(* Logix 5000 AddOnInstructionDefinition export Banner_Q20EAF_Param_v4; software revision 33.00; part 2 of 2 *)
(* tags used below, declared in another part *)
   Q20 : Banner_Q20EAF_v4;
   Port_Data : Banner_IOL_Port_v4;
   Port : DINT;
   Local_Control : DINT;
   Command_Being_Processed : BOOL;
   Update_Archive : BOOL;
   Index_Write_Inprocess : INT;
   Index_Write_Control : INT;
   Inprocess_Index : DINT;
(* Banner_Q20EAF_Param_v4, continued *)

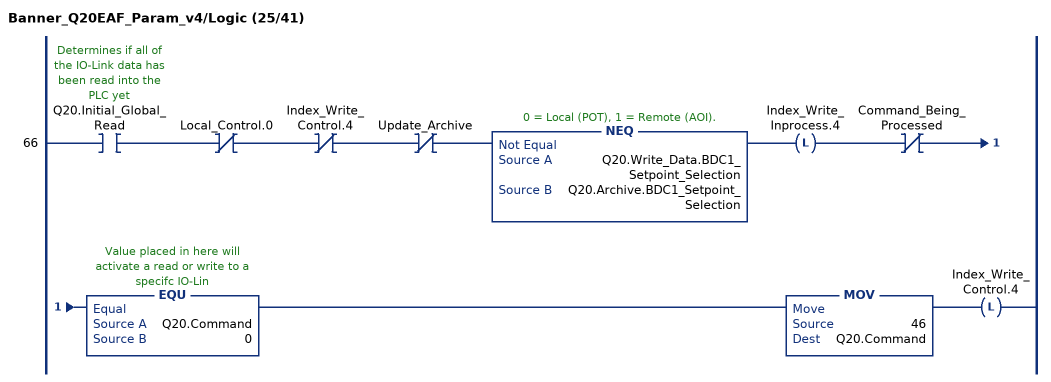
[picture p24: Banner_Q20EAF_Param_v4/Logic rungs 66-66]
   66: XIC(Q20.Initial_Global_Read)XIO(Local_Control.0)XIO(Index_Write_Control.4)XIO(Update_Archive)NEQ(Q20.Write_Data.BDC1_Setpoint_Selection,Q20.Archive.BDC1_Setpoint_Selection)OTL(Index_Write_Inprocess.4)XIO(Command_Being_Processed)EQU(Q20.Command,0)MOV(46,Q20.Command)OTL(Index_Write_Control.4);
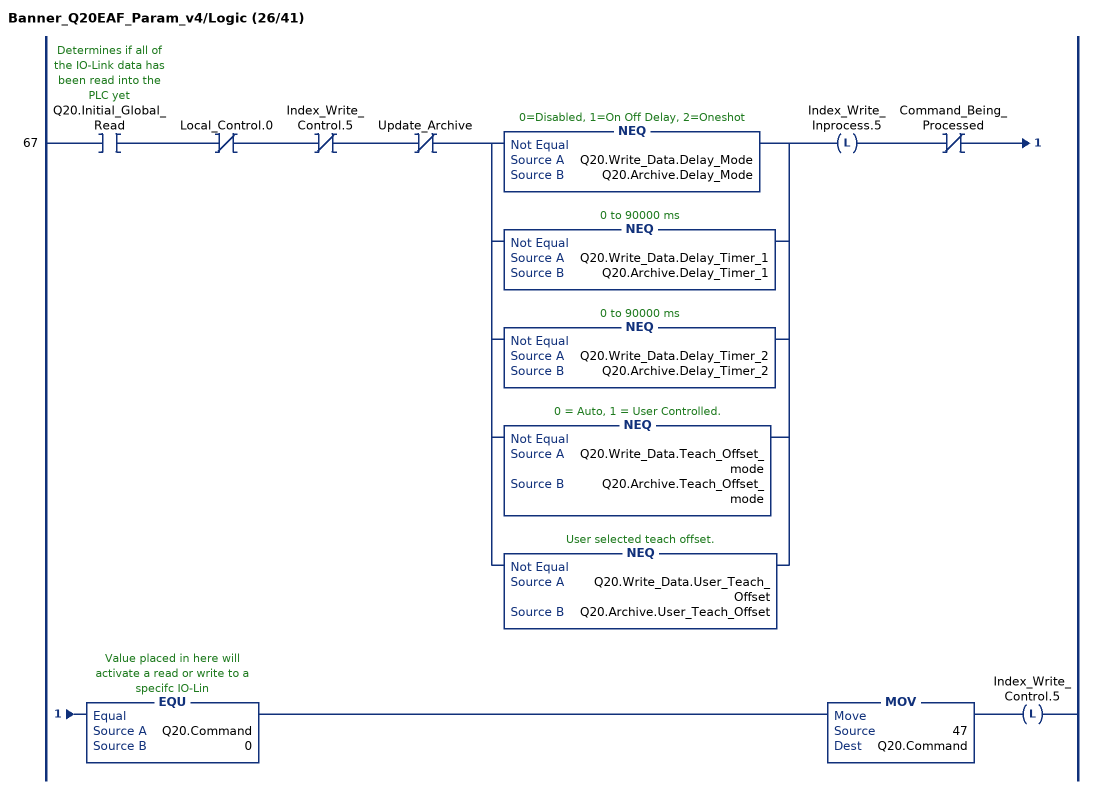
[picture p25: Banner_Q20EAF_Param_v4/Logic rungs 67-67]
   67: XIC(Q20.Initial_Global_Read)XIO(Local_Control.0)XIO(Index_Write_Control.5)XIO(Update_Archive)[NEQ(Q20.Write_Data.Delay_Mode,Q20.Archive.Delay_Mode) ,NEQ(Q20.Write_Data.Delay_Timer_1,Q20.Archive.Delay_Timer_1) ,NEQ(Q20.Write_Data.Delay_Timer_2,Q20.Archive.Delay_Timer_2) ,NEQ(Q20.Write_Data.Teach_Offset_mode,Q20.Archive.Teach_Offset_mode) ,NEQ(Q20.Write_Data.User_Teach_Offset,Q20.Archive.User_Teach_Offset) ]OTL(Index_Write_Inprocess.5)XIO(Command_Being_Processed)EQU(Q20.Command,0)MOV(47,Q20.Command)OTL(Index_Write_Control.5);
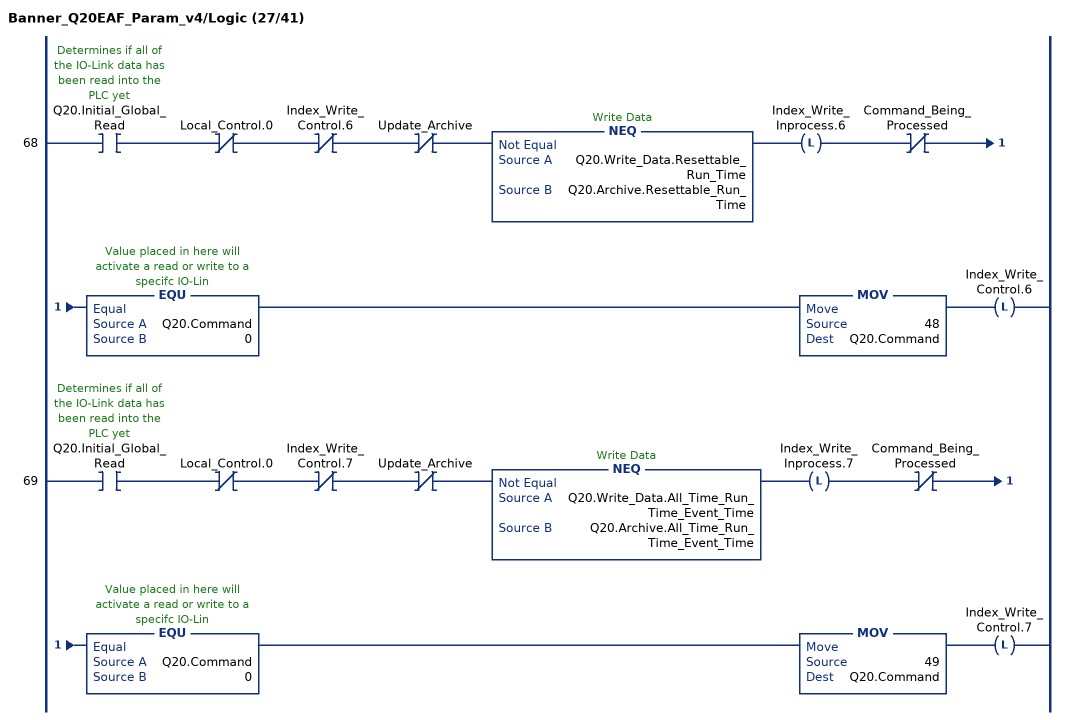
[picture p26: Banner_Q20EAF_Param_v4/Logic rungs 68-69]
   68: XIC(Q20.Initial_Global_Read)XIO(Local_Control.0)XIO(Index_Write_Control.6)XIO(Update_Archive)NEQ(Q20.Write_Data.Resettable_Run_Time,Q20.Archive.Resettable_Run_Time)OTL(Index_Write_Inprocess.6)XIO(Command_Being_Processed)EQU(Q20.Command,0)MOV(48,Q20.Command)OTL(Index_Write_Control.6);
   69: XIC(Q20.Initial_Global_Read)XIO(Local_Control.0)XIO(Index_Write_Control.7)XIO(Update_Archive)NEQ(Q20.Write_Data.All_Time_Run_Time_Event_Time,Q20.Archive.All_Time_Run_Time_Event_Time)OTL(Index_Write_Inprocess.7)XIO(Command_Being_Processed)EQU(Q20.Command,0)MOV(49,Q20.Command)OTL(Index_Write_Control.7);
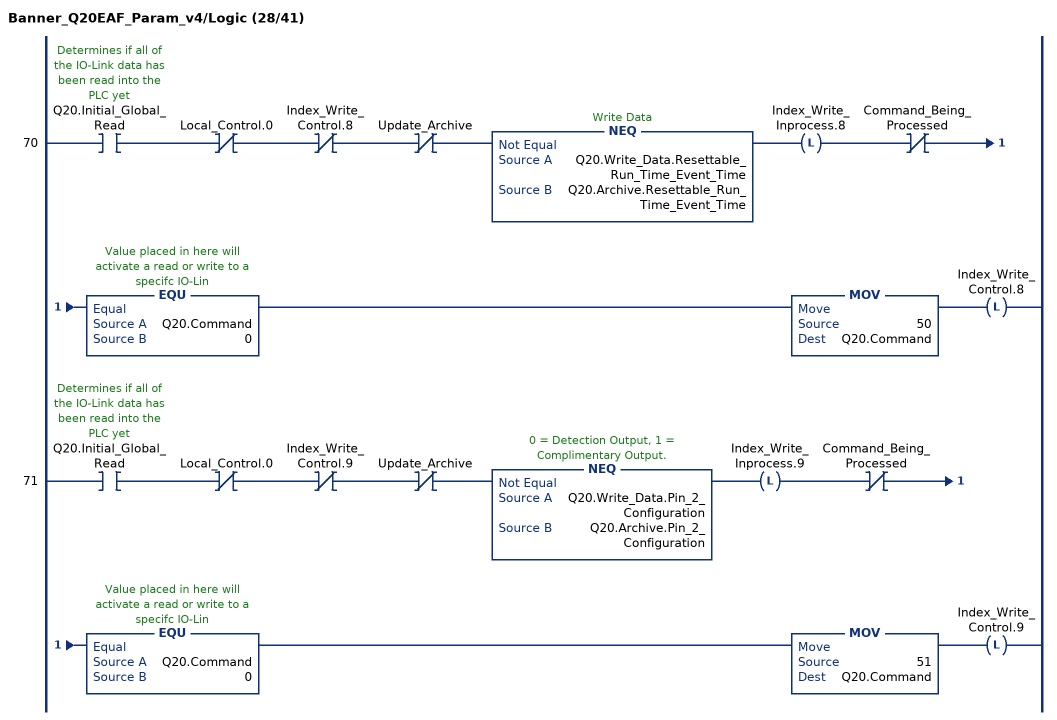
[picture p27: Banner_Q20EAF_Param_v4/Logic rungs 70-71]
   70: XIC(Q20.Initial_Global_Read)XIO(Local_Control.0)XIO(Index_Write_Control.8)XIO(Update_Archive)NEQ(Q20.Write_Data.Resettable_Run_Time_Event_Time,Q20.Archive.Resettable_Run_Time_Event_Time)OTL(Index_Write_Inprocess.8)XIO(Command_Being_Processed)EQU(Q20.Command,0)MOV(50,Q20.Command)OTL(Index_Write_Control.8);
   71: XIC(Q20.Initial_Global_Read)XIO(Local_Control.0)XIO(Index_Write_Control.9)XIO(Update_Archive)NEQ(Q20.Write_Data.Pin_2_Configuration,Q20.Archive.Pin_2_Configuration)OTL(Index_Write_Inprocess.9)XIO(Command_Being_Processed)EQU(Q20.Command,0)MOV(51,Q20.Command)OTL(Index_Write_Control.9);
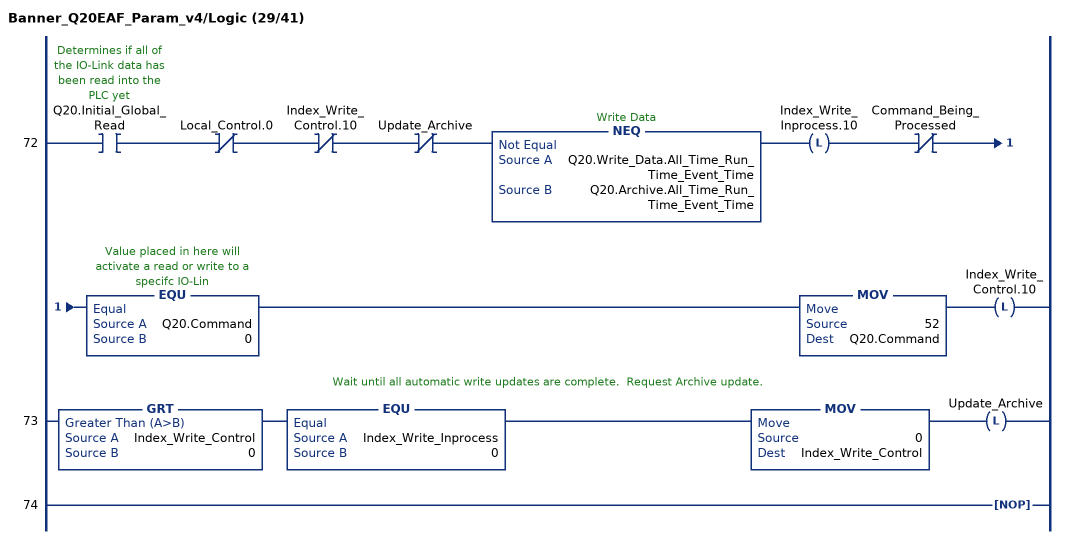
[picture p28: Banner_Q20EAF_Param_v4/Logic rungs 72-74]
   72: XIC(Q20.Initial_Global_Read)XIO(Local_Control.0)XIO(Index_Write_Control.10)XIO(Update_Archive)NEQ(Q20.Write_Data.All_Time_Run_Time_Event_Time,Q20.Archive.All_Time_Run_Time_Event_Time)OTL(Index_Write_Inprocess.10)XIO(Command_Being_Processed)EQU(Q20.Command,0)MOV(52,Q20.Command)OTL(Index_Write_Control.10);
   // Wait until all automatic write updates are complete.  Request Archive update.
   73: GRT(Index_Write_Control,0)EQU(Index_Write_Inprocess,0)MOV(0,Index_Write_Control)OTL(Update_Archive);
   74: NOP();
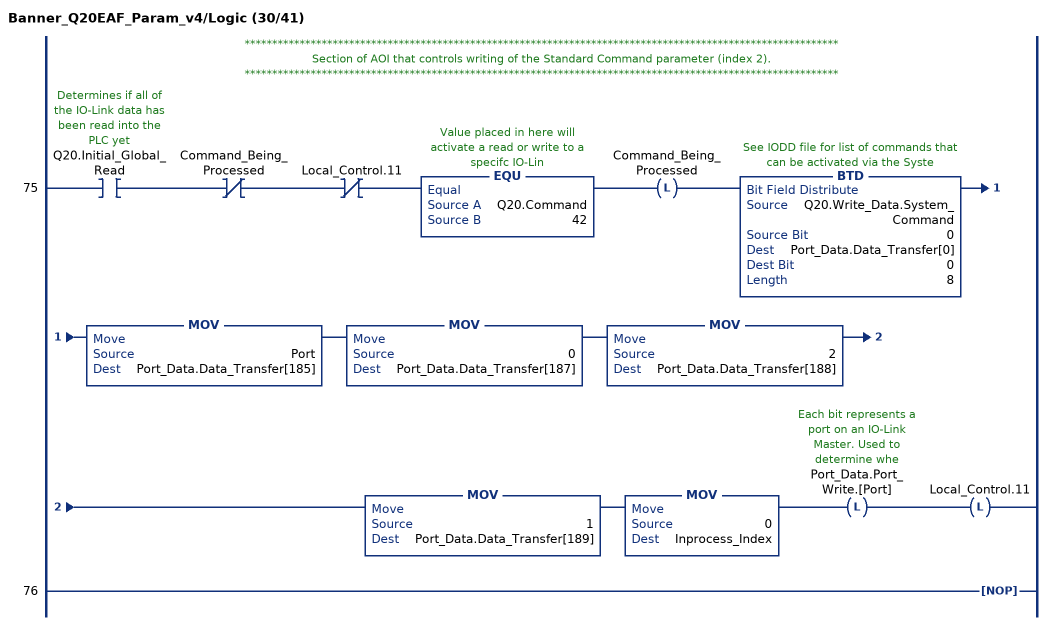
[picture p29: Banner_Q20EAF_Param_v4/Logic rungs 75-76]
   // ************************************************************************************************************
   // Section of AOI that controls writing of the Standard Command parameter (index 2).
   // ************************************************************************************************************
   75: XIC(Q20.Initial_Global_Read)XIO(Command_Being_Processed)XIO(Local_Control.11)EQU(Q20.Command,42)OTL(Command_Being_Processed)BTD(Q20.Write_Data.System_Command,0,Port_Data.Data_Transfer[0],0,8)MOV(Port,Port_Data.Data_Transfer[185])MOV(0,Port_Data.Data_Transfer[187])MOV(2,Port_Data.Data_Transfer[188])MOV(1,Port_Data.Data_Transfer[189])MOV(0,Inprocess_Index)OTL(Port_Data.Port_Write.[Port])OTL(Local_Control.11);
   76: NOP();
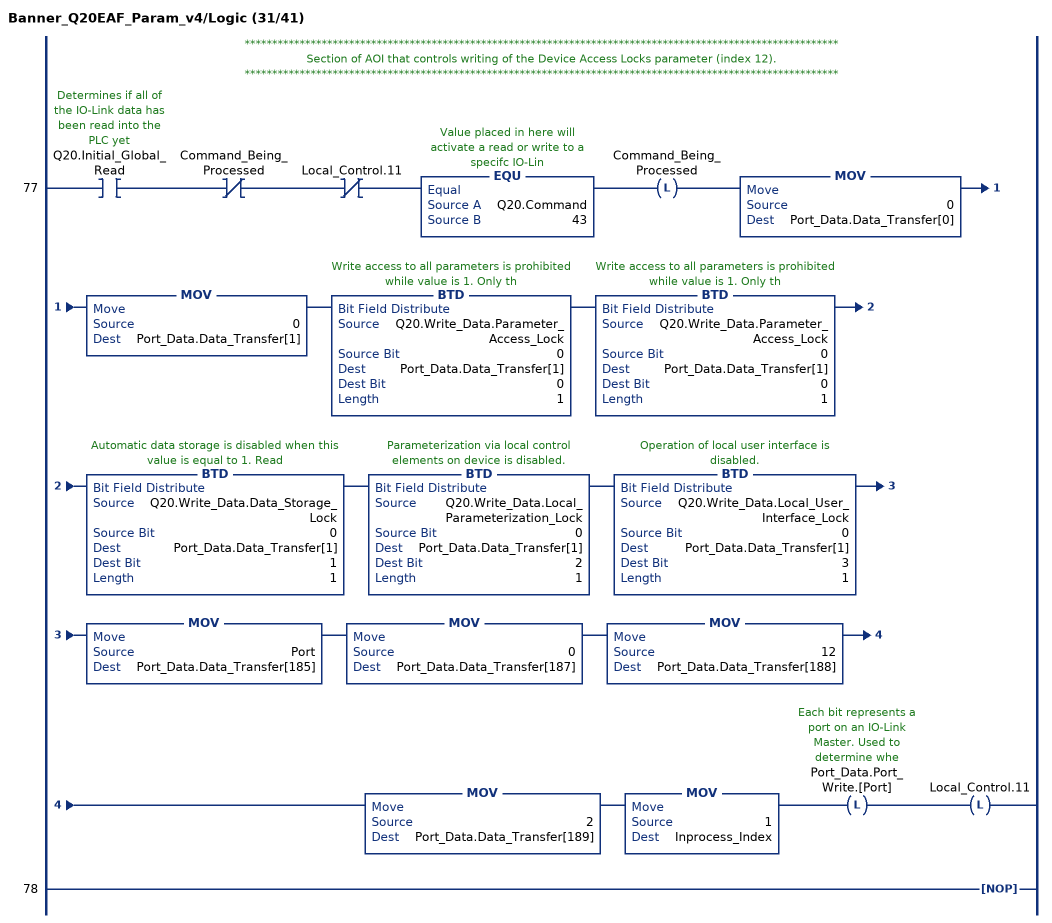
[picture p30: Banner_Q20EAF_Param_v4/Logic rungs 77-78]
   // ************************************************************************************************************
   // Section of AOI that controls writing of the Device Access Locks parameter (index 12).
   // ************************************************************************************************************
   77: XIC(Q20.Initial_Global_Read)XIO(Command_Being_Processed)XIO(Local_Control.11)EQU(Q20.Command,43)OTL(Command_Being_Processed)MOV(0,Port_Data.Data_Transfer[0])MOV(0,Port_Data.Data_Transfer[1])BTD(Q20.Write_Data.Parameter_Access_Lock,0,Port_Data.Data_Transfer[1],0,1)BTD(Q20.Write_Data.Parameter_Access_Lock,0,Port_Data.Data_Transfer[1],0,1)BTD(Q20.Write_Data.Data_Storage_Lock,0,Port_Data.Data_Transfer[1],1,1)BTD(Q20.Write_Data.Local_Parameterization_Lock,0,Port_Data.Data_Transfer[1],2,1)BTD(Q20.Write_Data.Local_User_Interface_Lock,0,Port_Data.Data_Transfer[1],3,1)MOV(Port,Port_Data.Data_Transfer[185])MOV(0,Port_Data.Data_Transfer[187])MOV(12,Port_Data.Data_Transfer[188])MOV(2,Port_Data.Data_Transfer[189])MOV(1,Inprocess_Index)OTL(Port_Data.Port_Write.[Port])OTL(Local_Control.11);
   78: NOP();
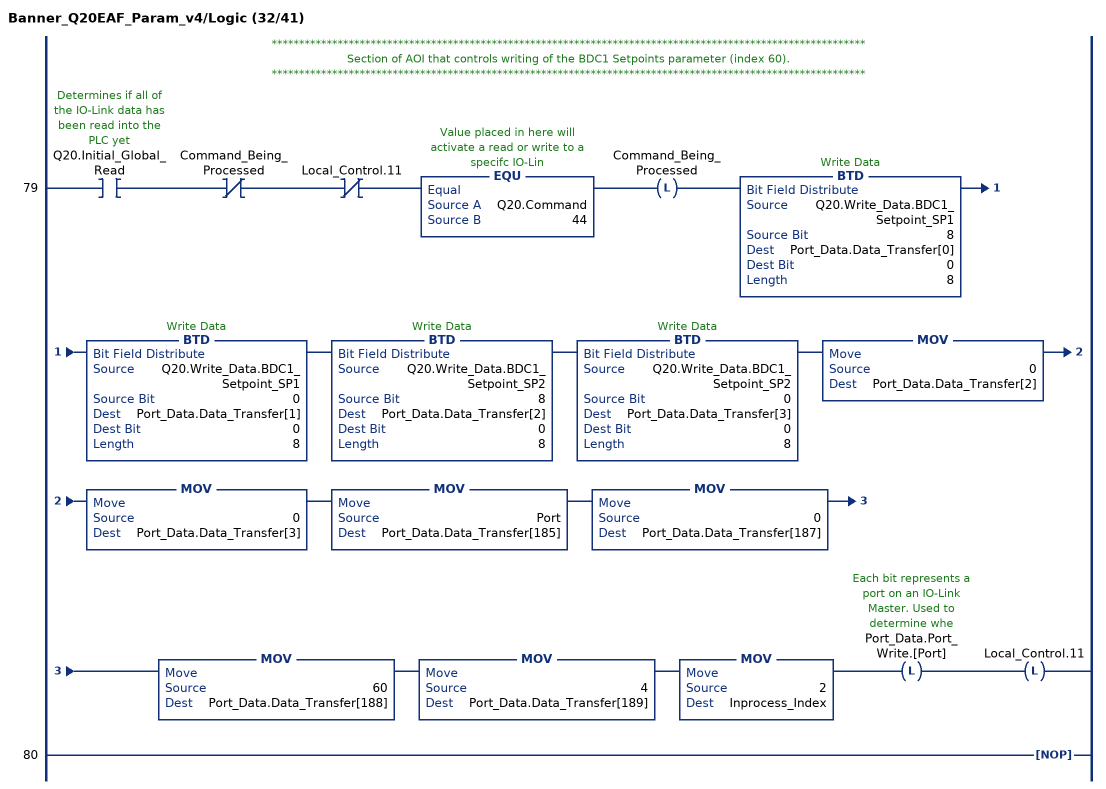
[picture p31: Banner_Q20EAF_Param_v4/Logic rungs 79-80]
   // ************************************************************************************************************
   // Section of AOI that controls writing of the BDC1 Setpoints parameter (index 60).
   // ************************************************************************************************************
   79: XIC(Q20.Initial_Global_Read)XIO(Command_Being_Processed)XIO(Local_Control.11)EQU(Q20.Command,44)OTL(Command_Being_Processed)BTD(Q20.Write_Data.BDC1_Setpoint_SP1,8,Port_Data.Data_Transfer[0],0,8)BTD(Q20.Write_Data.BDC1_Setpoint_SP1,0,Port_Data.Data_Transfer[1],0,8)BTD(Q20.Write_Data.BDC1_Setpoint_SP2,8,Port_Data.Data_Transfer[2],0,8)BTD(Q20.Write_Data.BDC1_Setpoint_SP2,0,Port_Data.Data_Transfer[3],0,8)MOV(0,Port_Data.Data_Transfer[2])MOV(0,Port_Data.Data_Transfer[3])MOV(Port,Port_Data.Data_Transfer[185])MOV(0,Port_Data.Data_Transfer[187])MOV(60,Port_Data.Data_Transfer[188])MOV(4,Port_Data.Data_Transfer[189])MOV(2,Inprocess_Index)OTL(Port_Data.Port_Write.[Port])OTL(Local_Control.11);
   80: NOP();
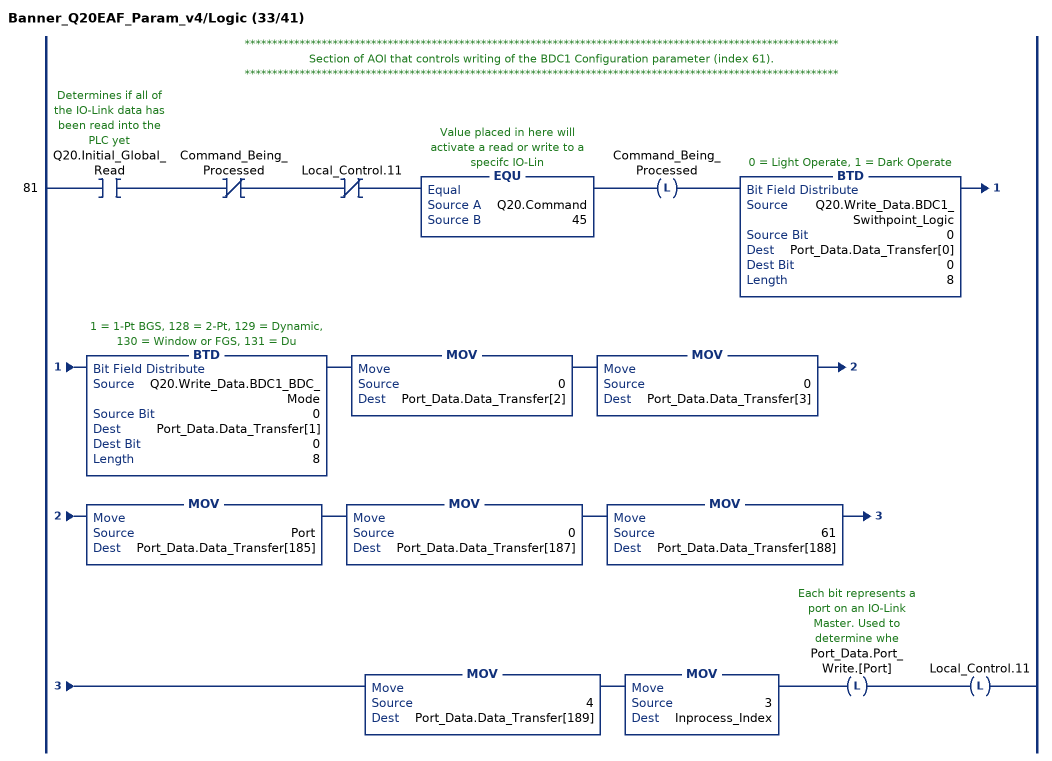
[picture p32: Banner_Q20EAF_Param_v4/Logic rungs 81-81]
   // ************************************************************************************************************
   // Section of AOI that controls writing of the BDC1 Configuration parameter (index 61).
   // ************************************************************************************************************
   81: XIC(Q20.Initial_Global_Read)XIO(Command_Being_Processed)XIO(Local_Control.11)EQU(Q20.Command,45)OTL(Command_Being_Processed)BTD(Q20.Write_Data.BDC1_Swithpoint_Logic,0,Port_Data.Data_Transfer[0],0,8)BTD(Q20.Write_Data.BDC1_BDC_Mode,0,Port_Data.Data_Transfer[1],0,8)MOV(0,Port_Data.Data_Transfer[2])MOV(0,Port_Data.Data_Transfer[3])MOV(Port,Port_Data.Data_Transfer[185])MOV(0,Port_Data.Data_Transfer[187])MOV(61,Port_Data.Data_Transfer[188])MOV(4,Port_Data.Data_Transfer[189])MOV(3,Inprocess_Index)OTL(Port_Data.Port_Write.[Port])OTL(Local_Control.11);
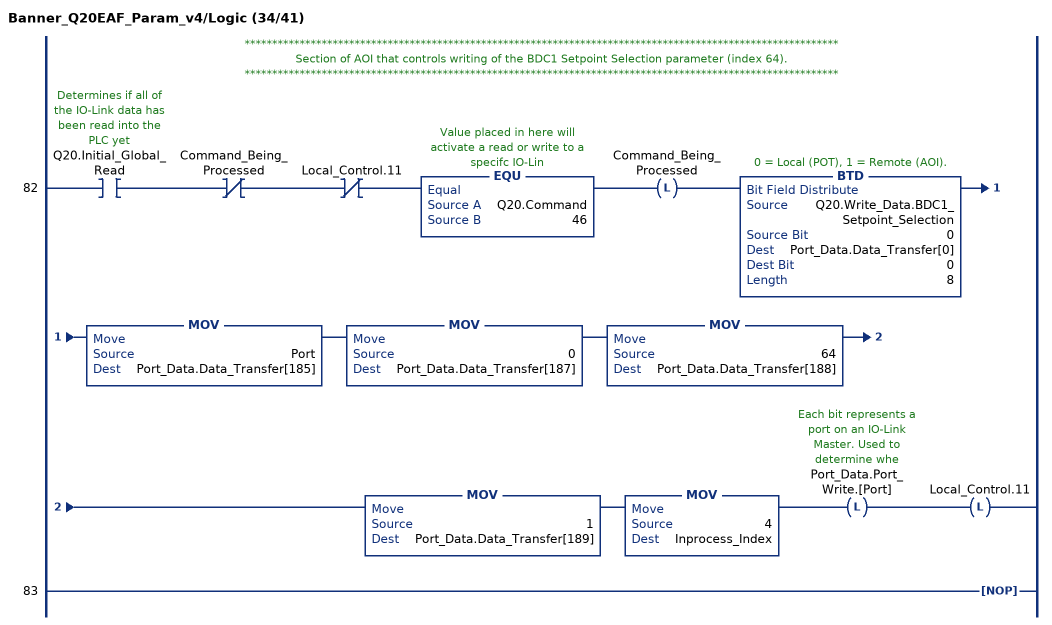
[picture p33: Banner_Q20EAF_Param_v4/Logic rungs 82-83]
   // ************************************************************************************************************
   // Section of AOI that controls writing of the BDC1 Setpoint Selection parameter (index 64).
   // ************************************************************************************************************
   82: XIC(Q20.Initial_Global_Read)XIO(Command_Being_Processed)XIO(Local_Control.11)EQU(Q20.Command,46)OTL(Command_Being_Processed)BTD(Q20.Write_Data.BDC1_Setpoint_Selection,0,Port_Data.Data_Transfer[0],0,8)MOV(Port,Port_Data.Data_Transfer[185])MOV(0,Port_Data.Data_Transfer[187])MOV(64,Port_Data.Data_Transfer[188])MOV(1,Port_Data.Data_Transfer[189])MOV(4,Inprocess_Index)OTL(Port_Data.Port_Write.[Port])OTL(Local_Control.11);
   83: NOP();
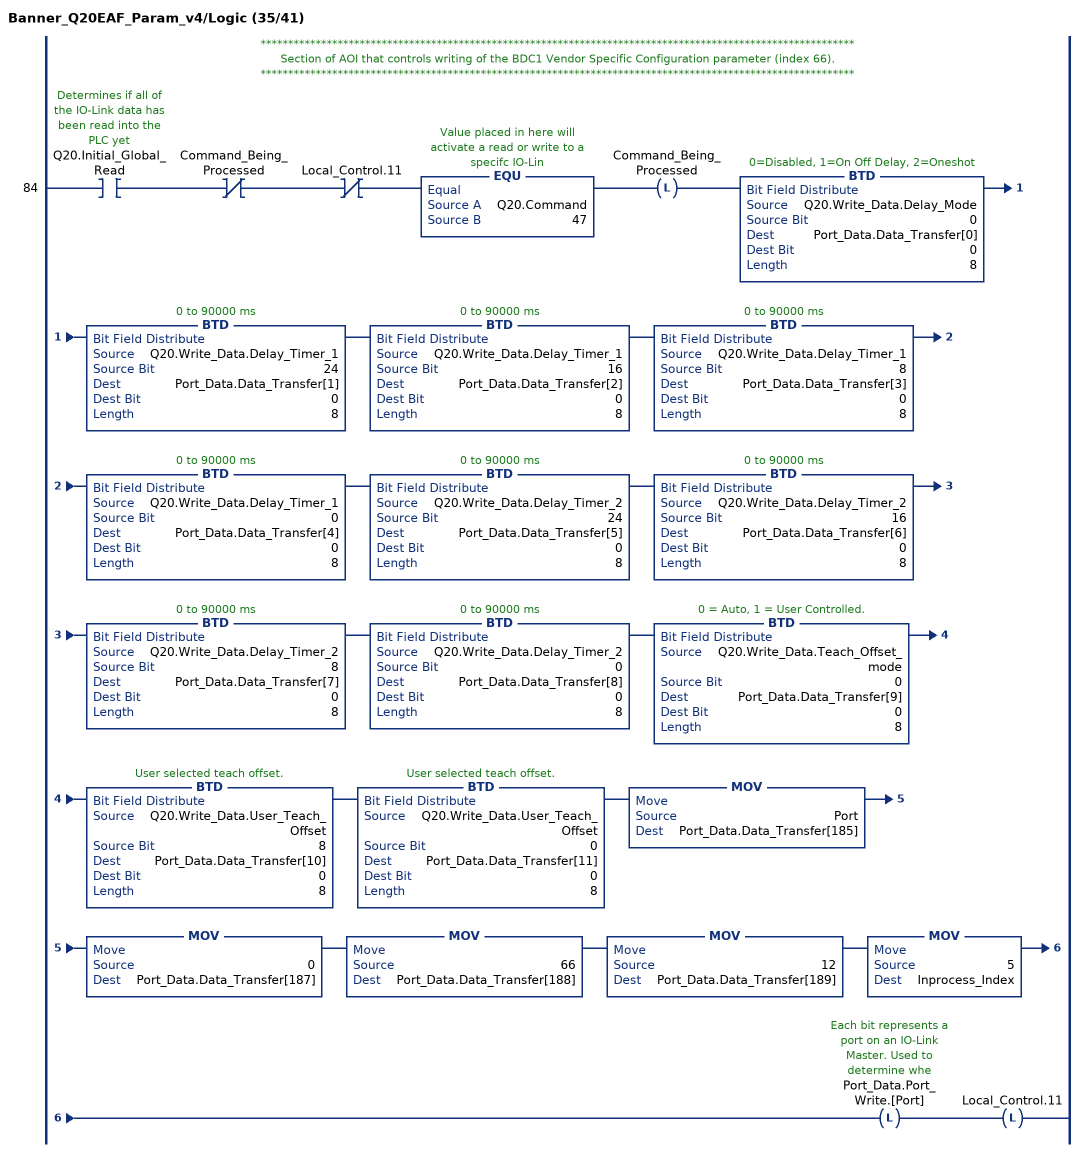
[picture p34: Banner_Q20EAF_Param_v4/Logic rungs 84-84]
   // ************************************************************************************************************
   // Section of AOI that controls writing of the BDC1 Vendor Specific Configuration parameter (index 66).
   // ************************************************************************************************************
   84: XIC(Q20.Initial_Global_Read)XIO(Command_Being_Processed)XIO(Local_Control.11)EQU(Q20.Command,47)OTL(Command_Being_Processed)BTD(Q20.Write_Data.Delay_Mode,0,Port_Data.Data_Transfer[0],0,8)BTD(Q20.Write_Data.Delay_Timer_1,24,Port_Data.Data_Transfer[1],0,8)BTD(Q20.Write_Data.Delay_Timer_1,16,Port_Data.Data_Transfer[2],0,8)BTD(Q20.Write_Data.Delay_Timer_1,8,Port_Data.Data_Transfer[3],0,8)BTD(Q20.Write_Data.Delay_Timer_1,0,Port_Data.Data_Transfer[4],0,8)BTD(Q20.Write_Data.Delay_Timer_2,24,Port_Data.Data_Transfer[5],0,8)BTD(Q20.Write_Data.Delay_Timer_2,16,Port_Data.Data_Transfer[6],0,8)BTD(Q20.Write_Data.Delay_Timer_2,8,Port_Data.Data_Transfer[7],0,8)BTD(Q20.Write_Data.Delay_Timer_2,0,Port_Data.Data_Transfer[8],0,8)BTD(Q20.Write_Data.Teach_Offset_mode,0,Port_Data.Data_Transfer[9],0,8)BTD(Q20.Write_Data.User_Teach_Offset,8,Port_Data.Data_Transfer[10],0,8)BTD(Q20.Write_Data.User_Teach_Offset,0,Port_Data.Data_Transfer[11],0,8)MOV(Port,Port_Data.Data_Transfer[185])MOV(0,Port_Data.Data_Transfer[187])MOV(66,Port_Data.Data_Transfer[188])MOV(12,Port_Data.Data_Transfer[189])MOV(5,Inprocess_Index)OTL(Port_Data.Port_Write.[Port])OTL(Local_Control.11);
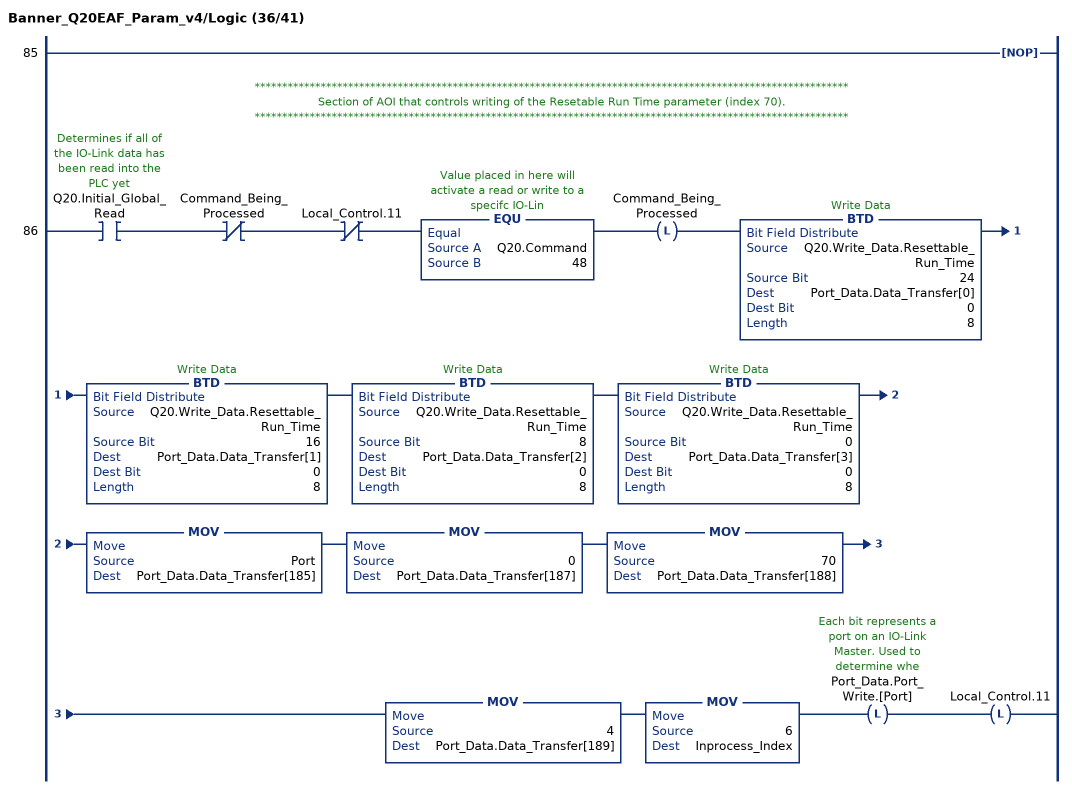
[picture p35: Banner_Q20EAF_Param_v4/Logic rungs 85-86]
   85: NOP();
   // ************************************************************************************************************
   // Section of AOI that controls writing of the Resetable Run Time parameter (index 70).
   // ************************************************************************************************************
   86: XIC(Q20.Initial_Global_Read)XIO(Command_Being_Processed)XIO(Local_Control.11)EQU(Q20.Command,48)OTL(Command_Being_Processed)BTD(Q20.Write_Data.Resettable_Run_Time,24,Port_Data.Data_Transfer[0],0,8)BTD(Q20.Write_Data.Resettable_Run_Time,16,Port_Data.Data_Transfer[1],0,8)BTD(Q20.Write_Data.Resettable_Run_Time,8,Port_Data.Data_Transfer[2],0,8)BTD(Q20.Write_Data.Resettable_Run_Time,0,Port_Data.Data_Transfer[3],0,8)MOV(Port,Port_Data.Data_Transfer[185])MOV(0,Port_Data.Data_Transfer[187])MOV(70,Port_Data.Data_Transfer[188])MOV(4,Port_Data.Data_Transfer[189])MOV(6,Inprocess_Index)OTL(Port_Data.Port_Write.[Port])OTL(Local_Control.11);
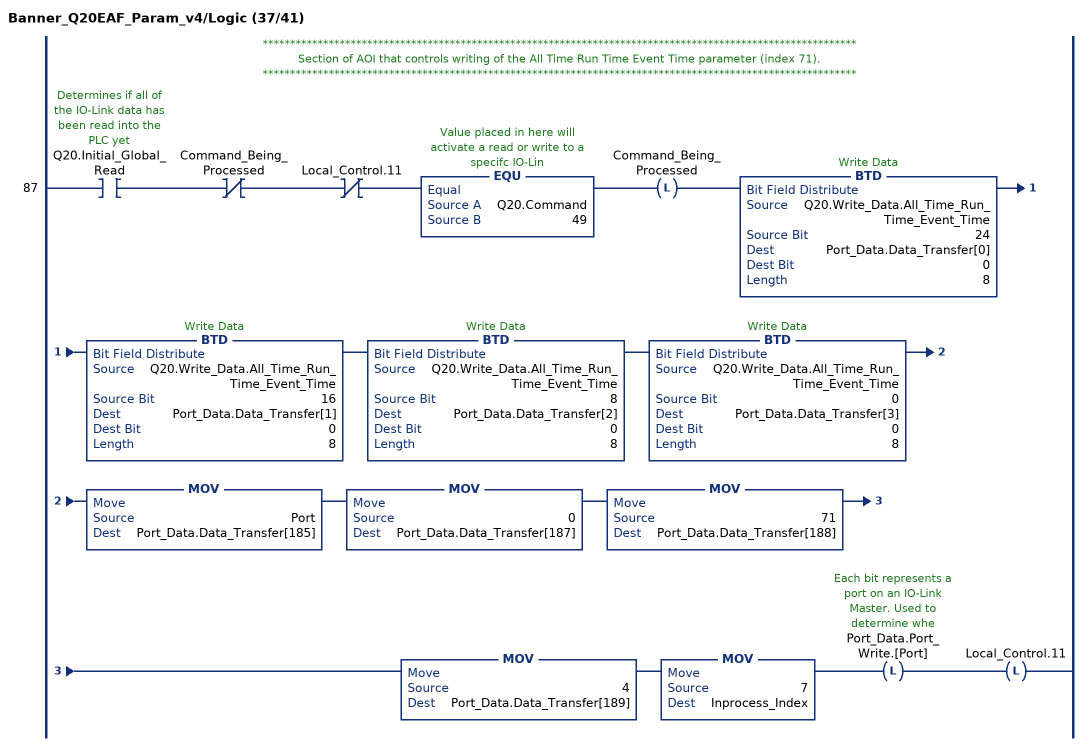
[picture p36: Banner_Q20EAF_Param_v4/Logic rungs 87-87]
   // ************************************************************************************************************
   // Section of AOI that controls writing of the All Time Run Time Event Time parameter (index 71).
   // ************************************************************************************************************
   87: XIC(Q20.Initial_Global_Read)XIO(Command_Being_Processed)XIO(Local_Control.11)EQU(Q20.Command,49)OTL(Command_Being_Processed)BTD(Q20.Write_Data.All_Time_Run_Time_Event_Time,24,Port_Data.Data_Transfer[0],0,8)BTD(Q20.Write_Data.All_Time_Run_Time_Event_Time,16,Port_Data.Data_Transfer[1],0,8)BTD(Q20.Write_Data.All_Time_Run_Time_Event_Time,8,Port_Data.Data_Transfer[2],0,8)BTD(Q20.Write_Data.All_Time_Run_Time_Event_Time,0,Port_Data.Data_Transfer[3],0,8)MOV(Port,Port_Data.Data_Transfer[185])MOV(0,Port_Data.Data_Transfer[187])MOV(71,Port_Data.Data_Transfer[188])MOV(4,Port_Data.Data_Transfer[189])MOV(7,Inprocess_Index)OTL(Port_Data.Port_Write.[Port])OTL(Local_Control.11);
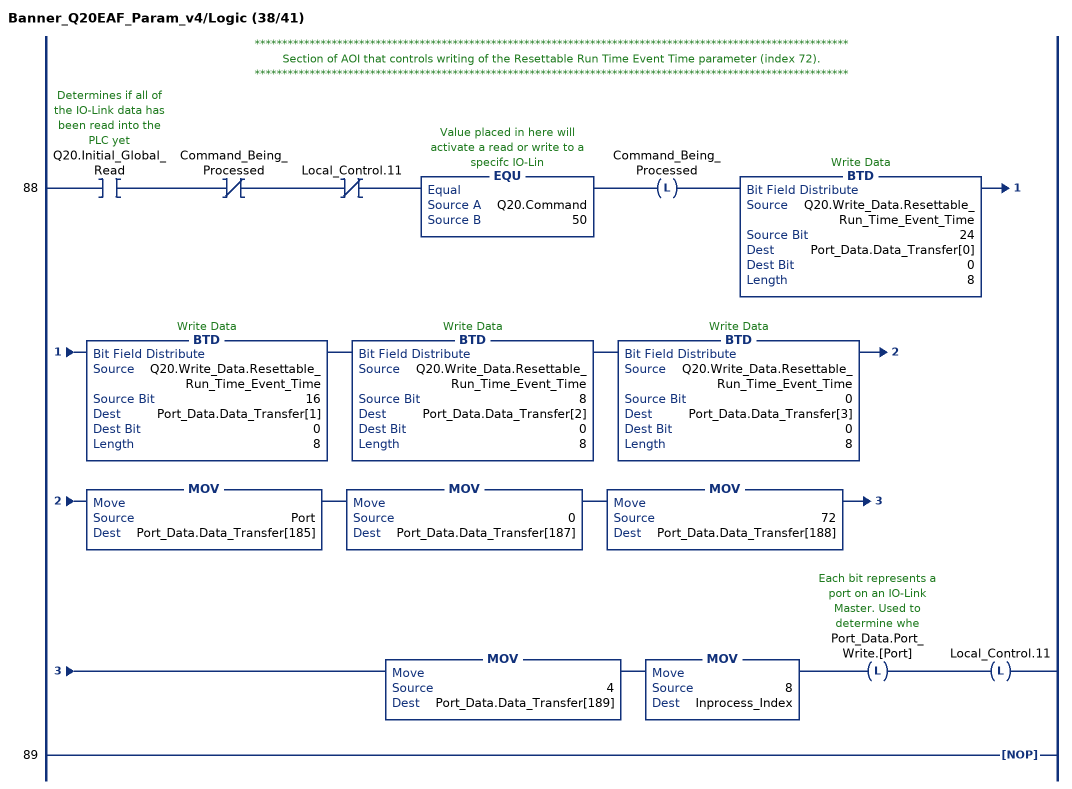
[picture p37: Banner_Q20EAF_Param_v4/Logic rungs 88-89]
   // ************************************************************************************************************
   // Section of AOI that controls writing of the Resettable Run Time Event Time parameter (index 72).
   // ************************************************************************************************************
   88: XIC(Q20.Initial_Global_Read)XIO(Command_Being_Processed)XIO(Local_Control.11)EQU(Q20.Command,50)OTL(Command_Being_Processed)BTD(Q20.Write_Data.Resettable_Run_Time_Event_Time,24,Port_Data.Data_Transfer[0],0,8)BTD(Q20.Write_Data.Resettable_Run_Time_Event_Time,16,Port_Data.Data_Transfer[1],0,8)BTD(Q20.Write_Data.Resettable_Run_Time_Event_Time,8,Port_Data.Data_Transfer[2],0,8)BTD(Q20.Write_Data.Resettable_Run_Time_Event_Time,0,Port_Data.Data_Transfer[3],0,8)MOV(Port,Port_Data.Data_Transfer[185])MOV(0,Port_Data.Data_Transfer[187])MOV(72,Port_Data.Data_Transfer[188])MOV(4,Port_Data.Data_Transfer[189])MOV(8,Inprocess_Index)OTL(Port_Data.Port_Write.[Port])OTL(Local_Control.11);
   89: NOP();
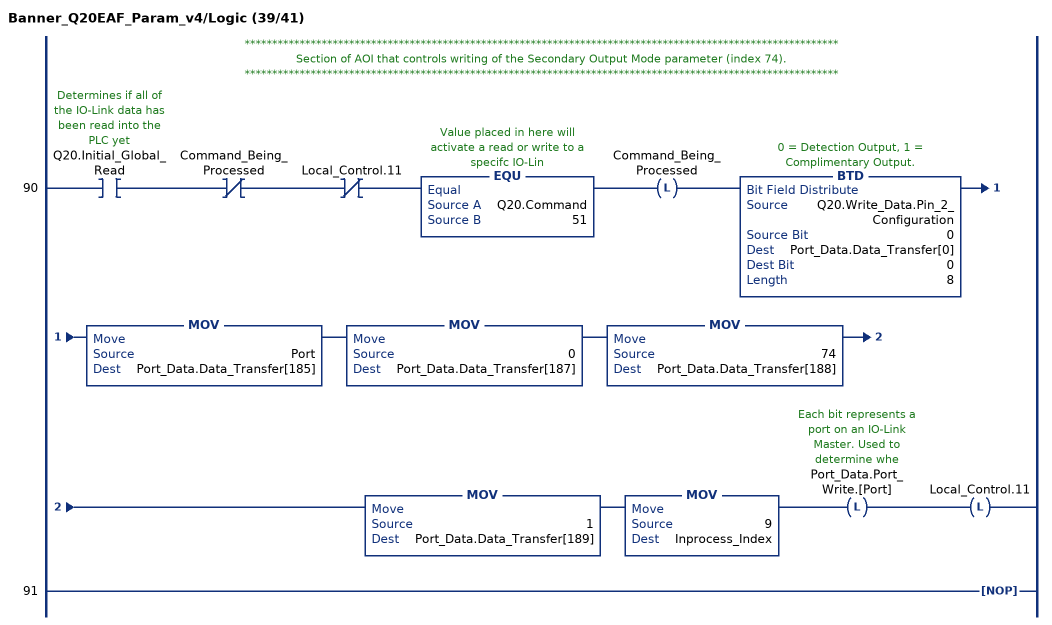
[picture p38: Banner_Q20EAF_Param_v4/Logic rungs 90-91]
   // ************************************************************************************************************
   // Section of AOI that controls writing of the Secondary Output Mode parameter (index 74).
   // ************************************************************************************************************
   90: XIC(Q20.Initial_Global_Read)XIO(Command_Being_Processed)XIO(Local_Control.11)EQU(Q20.Command,51)OTL(Command_Being_Processed)BTD(Q20.Write_Data.Pin_2_Configuration,0,Port_Data.Data_Transfer[0],0,8)MOV(Port,Port_Data.Data_Transfer[185])MOV(0,Port_Data.Data_Transfer[187])MOV(74,Port_Data.Data_Transfer[188])MOV(1,Port_Data.Data_Transfer[189])MOV(9,Inprocess_Index)OTL(Port_Data.Port_Write.[Port])OTL(Local_Control.11);
   91: NOP();
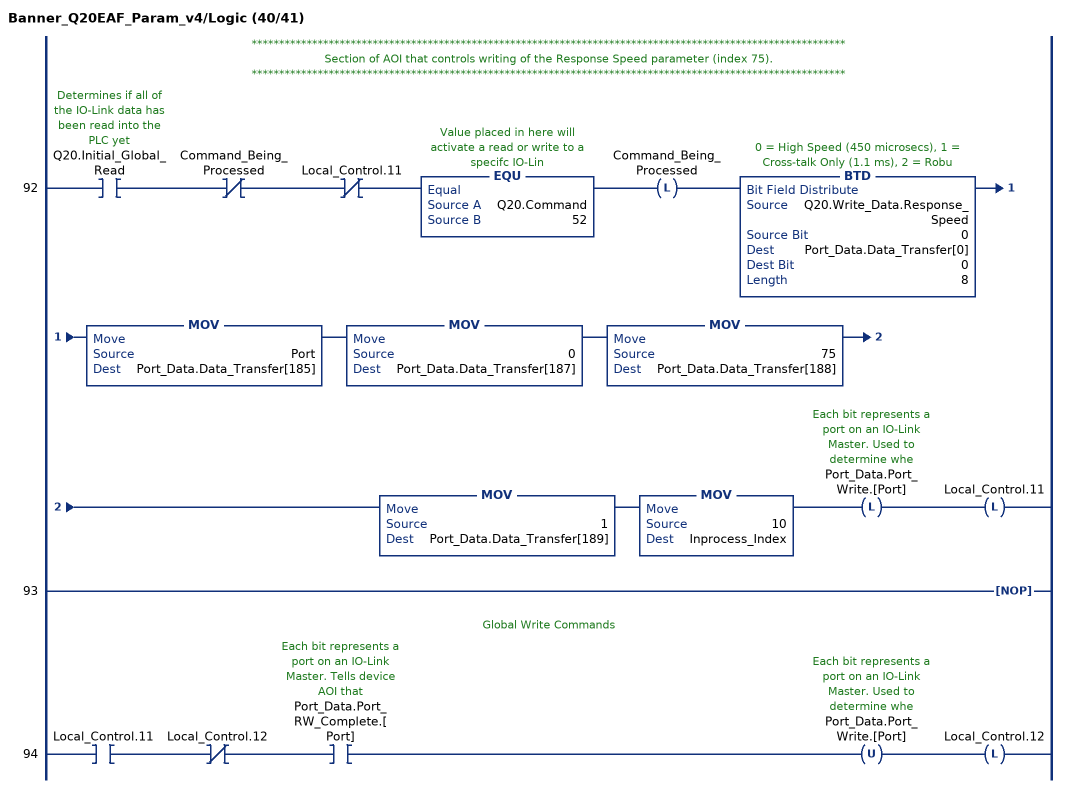
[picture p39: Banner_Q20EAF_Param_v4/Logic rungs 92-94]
   // ************************************************************************************************************
   // Section of AOI that controls writing of the Response Speed parameter (index 75).
   // ************************************************************************************************************
   92: XIC(Q20.Initial_Global_Read)XIO(Command_Being_Processed)XIO(Local_Control.11)EQU(Q20.Command,52)OTL(Command_Being_Processed)BTD(Q20.Write_Data.Response_Speed,0,Port_Data.Data_Transfer[0],0,8)MOV(Port,Port_Data.Data_Transfer[185])MOV(0,Port_Data.Data_Transfer[187])MOV(75,Port_Data.Data_Transfer[188])MOV(1,Port_Data.Data_Transfer[189])MOV(10,Inprocess_Index)OTL(Port_Data.Port_Write.[Port])OTL(Local_Control.11);
   93: NOP();
   // Global Write Commands
   94: XIC(Local_Control.11)XIO(Local_Control.12)XIC(Port_Data.Port_RW_Complete.[Port])OTU(Port_Data.Port_Write.[Port])OTL(Local_Control.12);
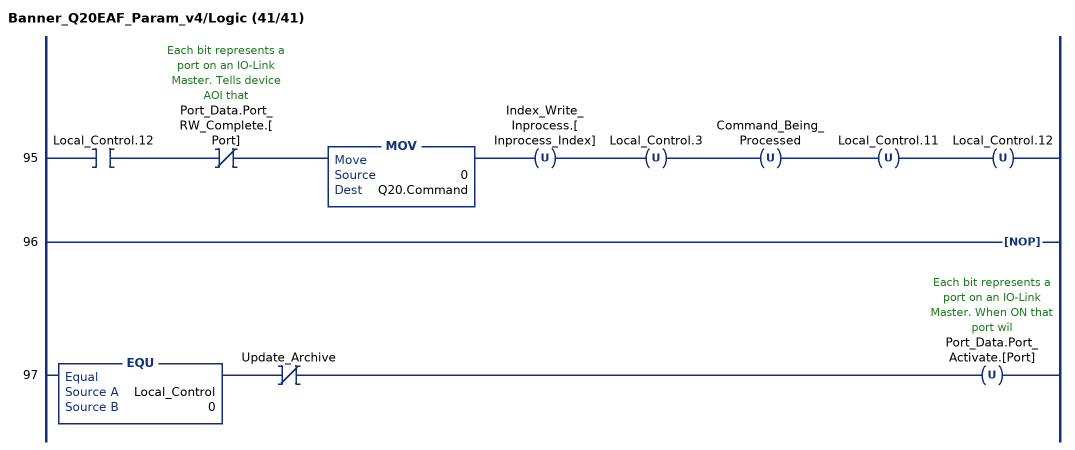
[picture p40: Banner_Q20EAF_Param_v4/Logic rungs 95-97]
   95: XIC(Local_Control.12)XIO(Port_Data.Port_RW_Complete.[Port])MOV(0,Q20.Command)OTU(Index_Write_Inprocess.[Inprocess_Index])OTU(Local_Control.3)OTU(Command_Being_Processed)OTU(Local_Control.11)OTU(Local_Control.12);
   96: NOP();
   97: EQU(Local_Control,0)XIO(Update_Archive)OTU(Port_Data.Port_Activate.[Port]);
END_ROUTINE
END_ADD_ON_INSTRUCTION
